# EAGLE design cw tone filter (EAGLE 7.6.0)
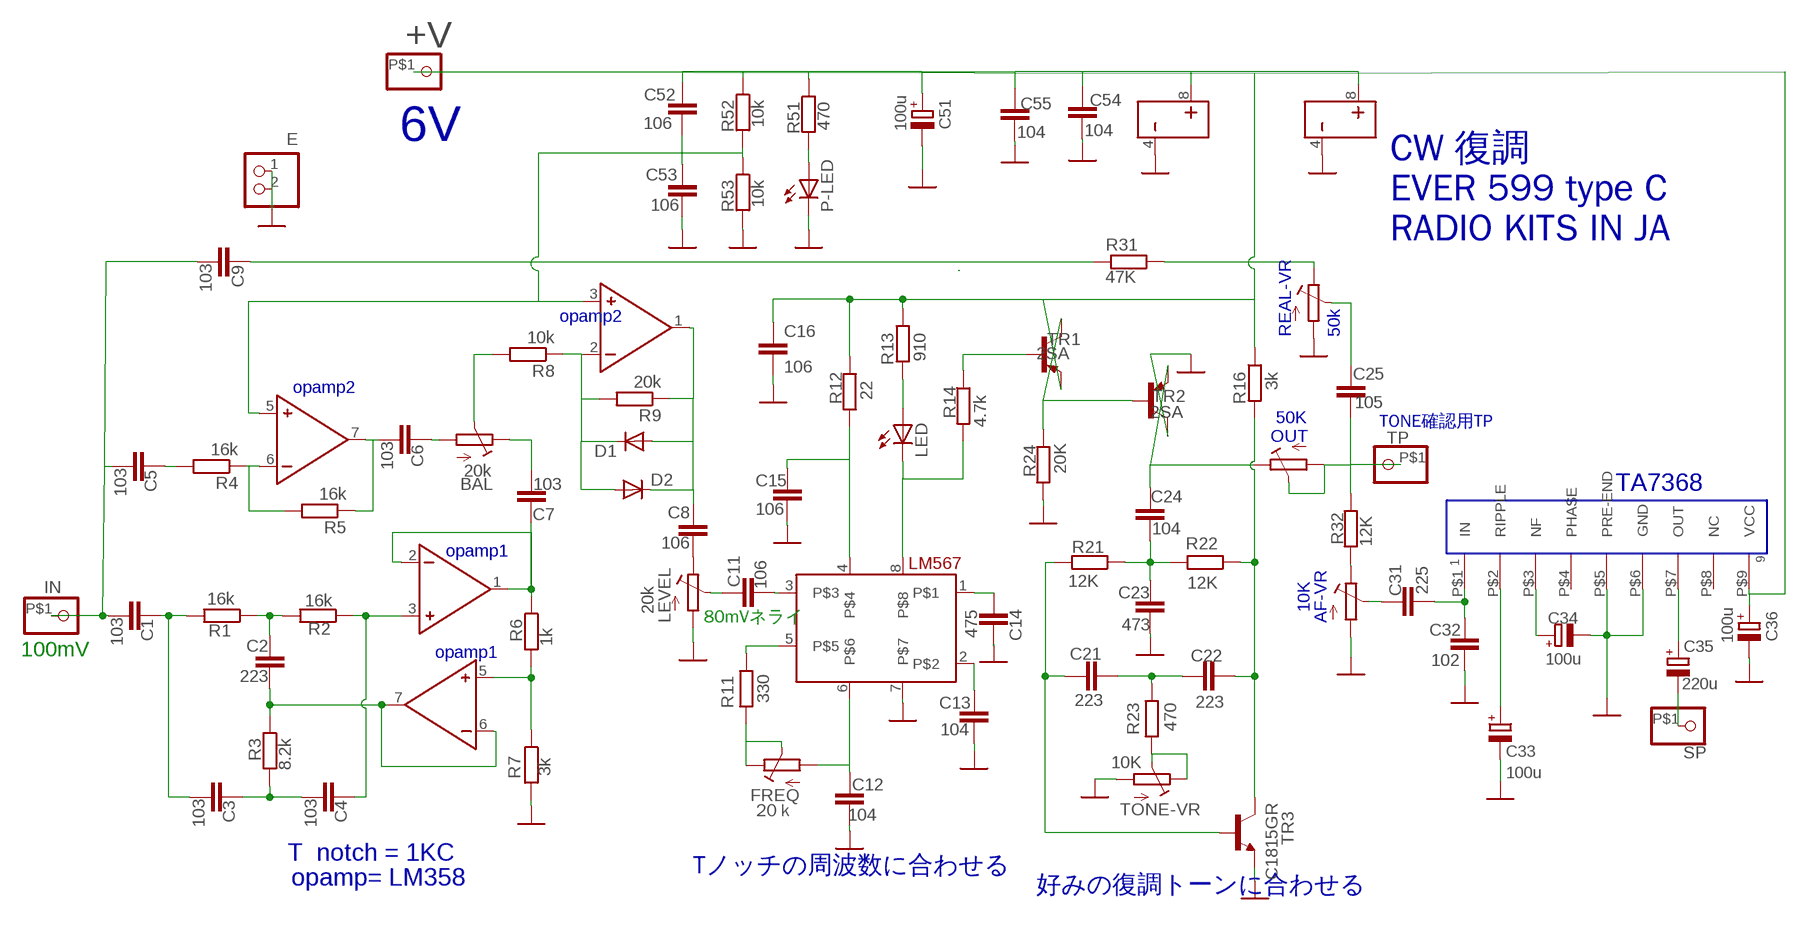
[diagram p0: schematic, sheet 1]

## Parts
+V  PINHD-1X1  [1X01]
AF-VR  10K  SINGLE-VR  [SINGLE-VR]
BAL  20k  R-TRIMM3296W  [RTRIM3296W]
C1  103  C-EU050-024X044  [C050-024X044]
C2  223  C-EU050-024X044  [C050-024X044]
C3  103  C-EU050-024X044  [C050-024X044]
C4  103  C-EU050-024X044  [C050-024X044]
C5  103  C-EU050-024X044  [C050-024X044]
C6  103  C-EU050-024X044  [C050-024X044]
C7  103  C-EU050-024X044  [C050-024X044]
C8  106  C-EU050-024X044  [C050-024X044]
C9  103  C-EU050-024X044  [C050-024X044]
C11  106  C-EU050-024X044  [C050-024X044]
C12  104  C-EU050-024X044  [C050-024X044]
C13  104  C-EU050-024X044  [C050-024X044]
C14  475  C-EU050-024X044  [C050-024X044]
C15  106  C-EU050-024X044  [C050-024X044]
C16  106  C-EU050-024X044  [C050-024X044]
C21  223  C-EU050-024X044  [C050-024X044]
C22  223  C-EU050-024X044  [C050-024X044]
C23  473  C-EU050-024X044  [C050-024X044]
C24  104  C-EU050-024X044  [C050-024X044]
C25  105  C-EU050-024X044  [C050-024X044]
C31  225  C-EU050-024X044  [C050-024X044]
C32  102  C-EU050-024X044  [C050-024X044]
C33  100u  CPOL-EUE2.5-6  [E2,5-6]
C34  100u  CPOL-EUE2.5-6  [E2,5-6]
C35  220u  CPOL-EUE2.5-6  [E2,5-6]
C36  100u  CPOL-EUE2.5-6  [E2,5-6]
C51  100u  CPOL-EUE2.5-6  [E2,5-6]
C52  106  C-EU050-024X044  [C050-024X044]
C53  106  C-EU050-024X044  [C050-024X044]
C54  104  C-EU050-024X044  [C050-024X044]
C55  104  C-EU050-024X044  [C050-024X044]
D1  DIODE-D-5  [D-5]
D2  DIODE-D-5  [D-5]
E  PINHD-1X2  [1X02]
FREQ  20ｋ  R-TRIMM3296W  [RTRIM3296W]
IN  PINHD-1X1  [1X01]
LED  LEDIRL80A  [IRL80A]
LEVEL  20k  R-TRIMM3296W  [RTRIM3296W]
LM567  LM567  [NE612]
OPAMP1  4558  [DIL08]
OPAMP2  4558  [DIL08]
OUT  50K  R-TRIMM3296W  [RTRIM3296W]
P-LED  LEDIRL80A  [IRL80A]
R1  16k  R-EU_0204/5  [0204/5]
R2  16k  R-EU_0204/5  [0204/5]
R3  8.2k  R-EU_0204/5  [0204/5]
R4  16k  R-EU_0204/5  [0204/5]
R5  16k  R-EU_0204/5  [0204/5]
R6  1k  R-EU_0204/5  [0204/5]
R7  3k  R-EU_0204/5  [0204/5]
R8  10k  R-EU_0204/5  [0204/5]
R9  20k  R-EU_0204/5  [0204/5]
R11  330  R-EU_0204/5  [0204/5]
R12  22  R-EU_0204/5  [0204/5]
R13  910  R-EU_0204/5  [0204/5]
R14  4.7k  R-EU_0204/5  [0204/5]
R16  3k  R-EU_0204/5  [0204/5]
R21  12K  R-EU_0204/5  [0204/5]
R22  12K  R-EU_0204/5  [0204/5]
R23  470  R-EU_0204/5  [0204/5]
R24  20K  R-EU_0204/5  [0204/5]
R31  47K  R-EU_0204/5  [0204/5]
R32  12K  R-EU_0204/5  [0204/5]
R51  470  R-EU_0204/5  [0204/5]
R52  10k  R-EU_0204/5  [0204/5]
R53  10k  R-EU_0204/5  [0204/5]
REAL-VR  50k  R-TRIMM3296W  [RTRIM3296W]
SP  PINHD-1X1  [1X01]
TA7368  TA7368P  [TA7368P]
TONE-VR  10K  R-TRIMM3296W  [RTRIM3296W]
TP  PINHD-1X1  [1X01]
TR1  2SA  [TO92-ECB]
TR2  2SA  [TO92-ECB]
TR3  C1815GR  2SC1815  [TO92-ECB]

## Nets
9V: +V.P$1 C16.1 C36.+ C51.+ C52.1 C54.2 C55.2 OPAMP1.8 OPAMP2.8 R12.1 R13.1 R16.1 R51.1 R52.1 TA7368.P$9(VCC) TR1.E
GND: AF-VR.P$3(E) C12.2 C13.2 C14.1 C15.2 C16.2 C23.2 C32.2 C33.- C34.- C36.- C51.- C53.2 C54.1 C55.1 E.1 E.2 LEVEL.1(E) LM567.7 OPAMP1.4 OPAMP2.4 P-LED.K(C) R7.2 R24.2 R53.2 REAL-VR.1(E) TA7368.P$5(PRE-END) TA7368.P$6(GND) TONE-VR.1(E) TR2.C TR3.E
N$1: C8.2 LEVEL.3(A)
N$2: C52.2 C53.1 OPAMP2.3 OPAMP2.5 R52.2 R53.1
N$3: C25.2 REAL-VR.2(S)
N$4: C11.1 LM567.3
N$5: C2.1 R1.1 R2.2
N$6: C13.1 LM567.2
N$7: C3.2 C4.1 R3.2
N$8: C14.2 LM567.1
N$9: C1.2 C3.1 R1.2
N$10: C1.1 C5.1 C9.1 IN.P$1
N$11: LM567.5 R11.1
N$12: C24.1 OUT.3(A) TR2.E
N$13: C31.2 C32.1 TA7368.P$1(IN)
N$14: C35.- SP.P$1
N$15: AF-VR.P$2(S) C31.1
N$16: C35.+ TA7368.P$7(OUT)
N$18: C4.2 OPAMP1.3 R2.1
N$19: AF-VR.P$1(A) R32.2
N$20: C22.2 R16.2 R22.1 TR3.C
N$21: R31.1 REAL-VR.3(A)
N$22: C7.1 OPAMP1.1 OPAMP1.2 R6.1
N$23: OPAMP1.5 R6.2 R7.1
N$24: LED.A R13.2
N$25: C2.2 OPAMP1.6 OPAMP1.7 R3.1
N$27: BAL.1(E) C6.2
N$28: C6.1 OPAMP2.7 R5.1
N$29: C5.2 R4.2
N$30: OPAMP2.6 R4.1 R5.2
N$31: BAL.3(A) C7.2
N$32: BAL.2(S) R8.2
N$33: D1.C D2.A OPAMP2.2 R8.1 R9.2
N$34: C8.1 D1.A D2.C OPAMP2.1 R9.1
N$35: C12.1 FREQ.1(E) LM567.6
N$36: R24.1 TR1.C TR2.B
N$38: R23.1 TONE-VR.2(S) TONE-VR.3(A)
N$39: LED.K(C) LM567.8 R14.2
N$41: C25.1 OUT.1(E) OUT.2(S) R32.1 TP.P$1
N$42: C9.2 R31.2
N$43: C15.1 LM567.4 R12.2
N$44: C21.2 C22.1 R23.2
N$45: C21.1 R21.2 TR3.B
N$46: C11.2 LEVEL.2(S)
N$47: C23.1 C24.2 R21.1 R22.2
N$49: C34.+ TA7368.P$3(NF)
N$50: C33.+ TA7368.P$2(RIPPLE)
N$52: R14.1 TR1.B
N$53: FREQ.2(S) FREQ.3(A) R11.2
N$59: P-LED.A R51.2
Unconnected: TA7368.P$4(PHASE) TA7368.P$8(NC)

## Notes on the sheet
- 6V
- CW 復調　
  EVER 599 type C
  RADIO KITS IN JA
- opamp2
- opamp2
- TONE確認用TP
- opamp1
- 80mVネライ
- 100mV | opamp1
- T  notch = 1KC
- Tノッチの周波数に合わせる
- opamp= LM358
- 好みの復調トーンに合わせる

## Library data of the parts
+V IN SP TP = pinhead:PINHD-1X1: PIN HEADER
AF-VR = resistor:SINGLE-VR
BAL FREQ LEVEL OUT REAL-VR TONE-VR = resistor:R-TRIMM: Trimm resistor
C1-C9 C11-C16 C21-C25 C31 C32 C52-C55 = resistor:C-EU: CAPACITOR, European symbol
C33-C36 C51 = resistor:CPOL-EU: POLARIZED CAPACITOR, European symbol
D1 D2 = diode:DIODE-: DIODE
E = pinhead:PINHD-1X2: PIN HEADER
LED P-LED = led:LED: LED
LM567 = ssm2166 :LM567
OPAMP1 OPAMP2 = ic-package:4558
R1-R9 R11-R14 R16 R21-R24 R31 R32 R51-R53 = resistor:R-EU_: RESISTOR, European symbol
TA7368 = lc7265:TA7368P
TR1 TR2 = transistor:2SA
TR3 = transistor:2SC1815: NPN EPITAXIAL TRANSISTOR Source: TOSHIBA .. 2SC1815 1.pdf

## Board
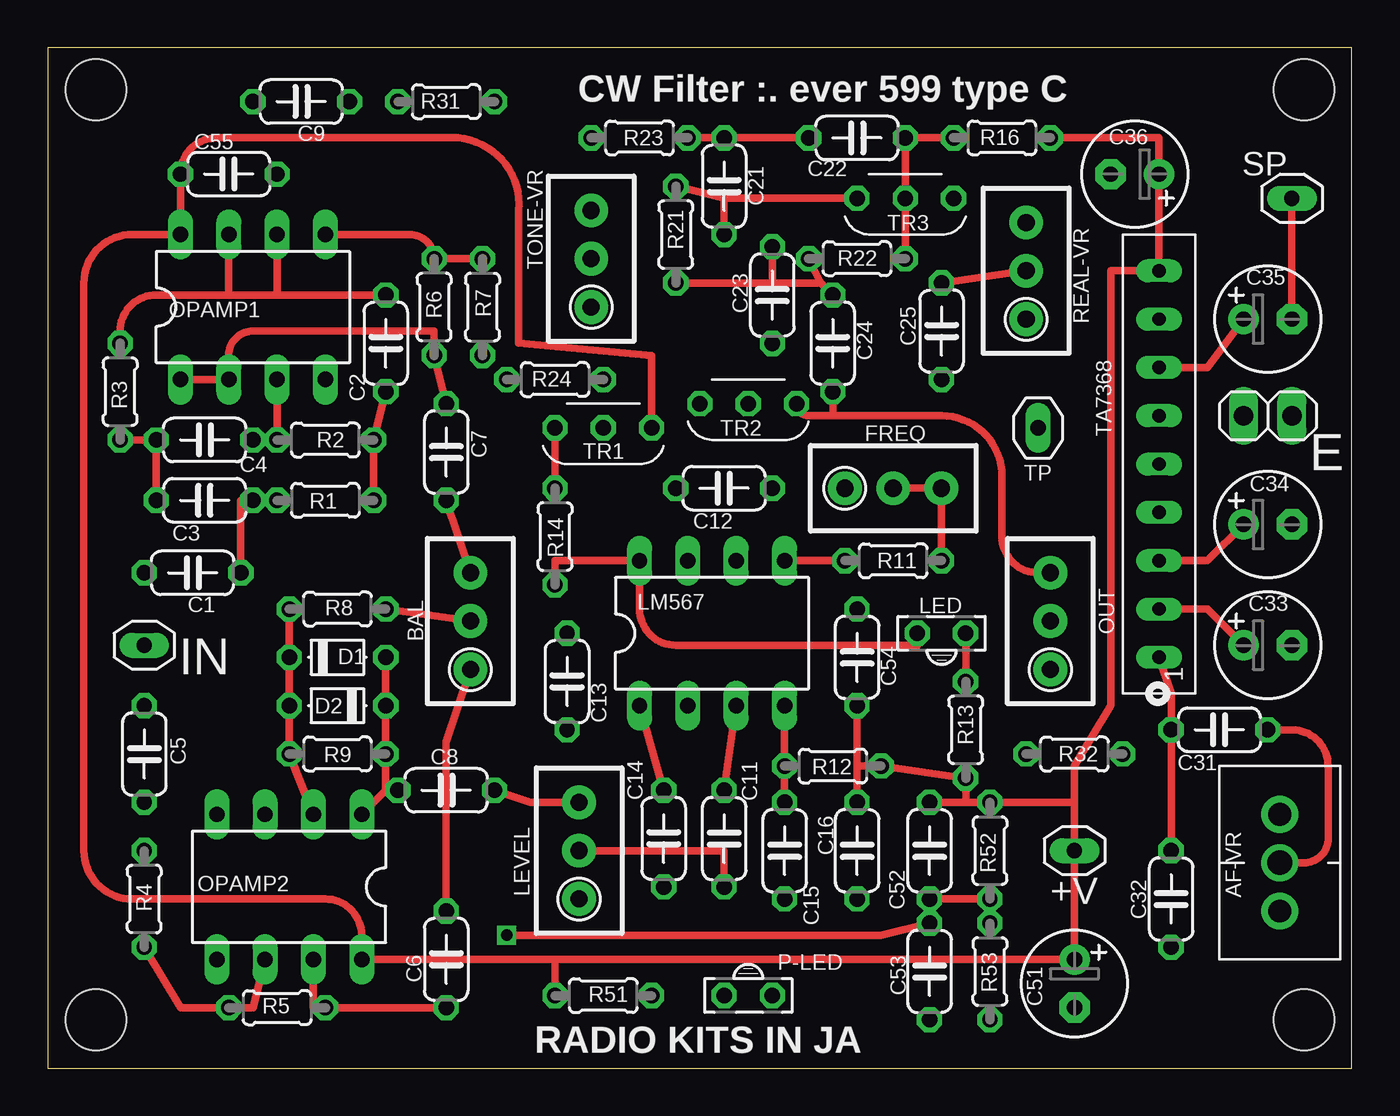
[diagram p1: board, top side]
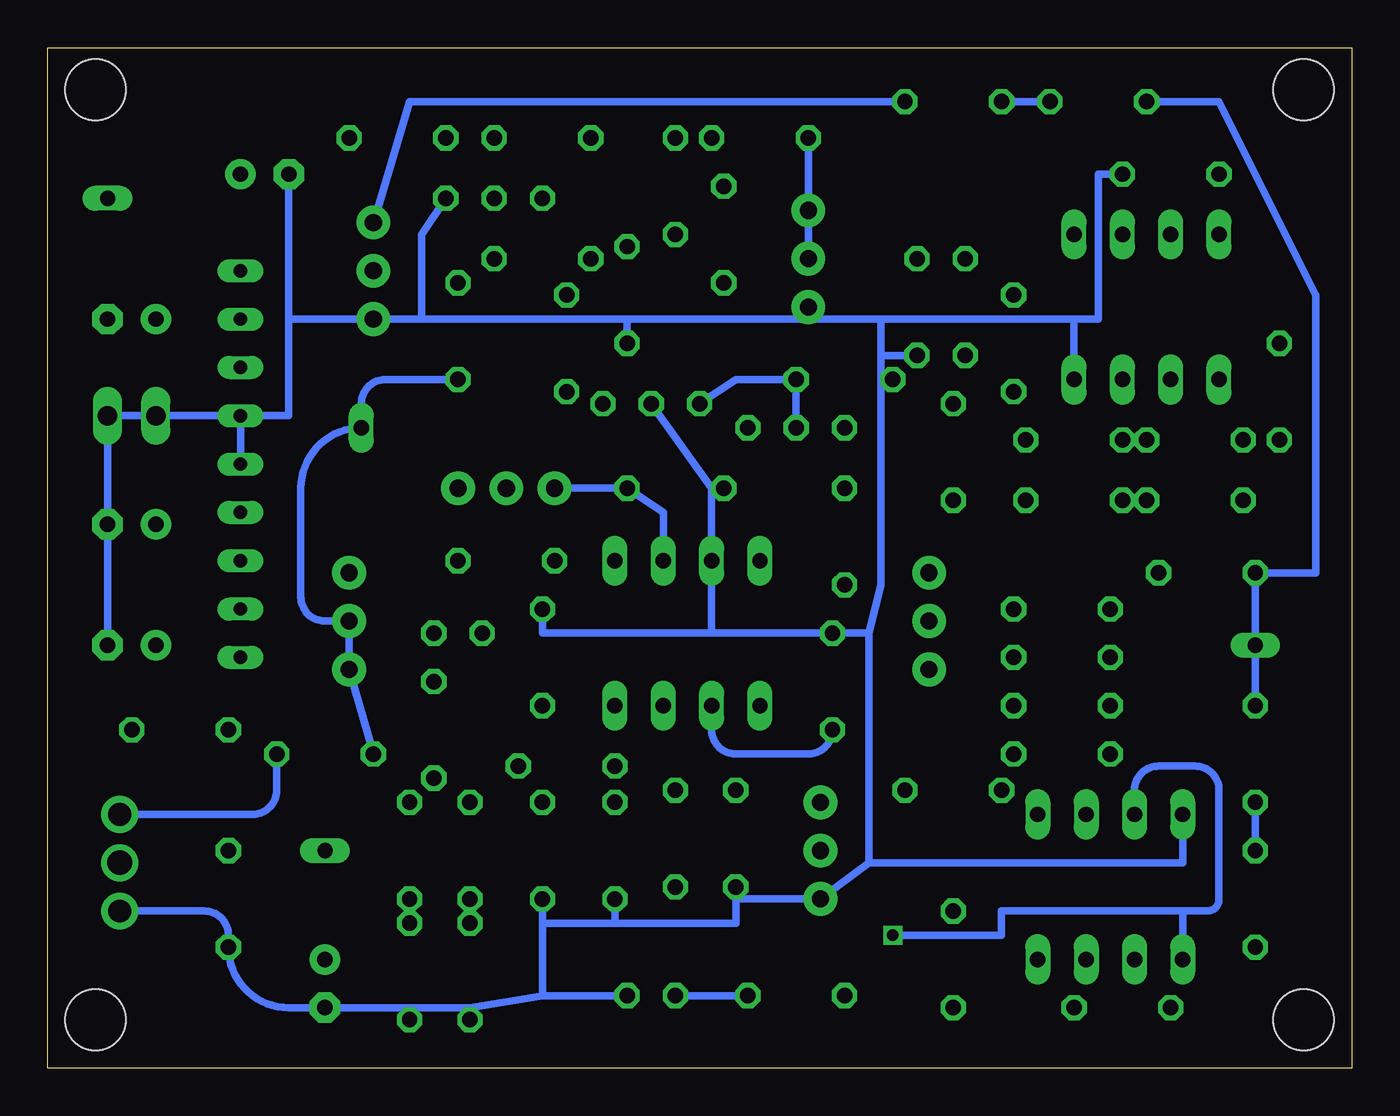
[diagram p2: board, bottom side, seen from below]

Size 68.56 x 53.65 mm. Coordinates in mm from the lower left corner, seen from the top.
Outline: 0,0 68.56,0 68.56,53.65 0,53.65 0,0
Copper layers (1*16): Top 0.035mm / dielectric 1.5mm / Bottom 0.035mm
Design rules "default": minimum track width 10mil, minimum drill 24mil, track to track 8mil, track to pad 8mil, pad to pad 8mil, via to via 8mil, smd to smd 8mil, copper to edge 40mil, drill to drill 8mil, minimum pad ring 10mil, minimum via ring 8mil, stop-mask expansion 4mil, vias tented up to drill 0mil, thermal gap 10mil
Holes 3.2 mm at 66.04,2.54 2.54,51.44 2.54,2.54 66.04,51.44

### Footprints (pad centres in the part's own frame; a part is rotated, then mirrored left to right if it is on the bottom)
1X01 = drill 0.8 long: P$1 0,0
SINGLE-VR = drill 1.2 pad 1.93: P$1 0.635,2.54; P$3 0.635,-2.54 | drill 1.3 pad 1.93: P$2 0.635,0
RTRIM3296W = drill 0.9 pad 1.778: 1 0,-2.54; 2 0,0; 3 0,2.54
C050-024X044 = drill 0.813 octagon: 1 -2.54,0; 2 2.54,0
E2,5-6 = drill 0.813 pad 1.6: + -1.27,0 | drill 0.813 pad 1.6 octagon: - 1.27,0
D-5 = drill 0.813 octagon: A 2.54,0; C -2.54,0
1X02 = drill 1.016 long: 1 -1.27,0; 2 1.27,0
IRL80A = drill 0.813 octagon: A 0,-1.27; K 0,1.27
NE612 = drill 0.813 long: 1 1.27,-3.81; 2 3.81,-3.81; 3 6.35,-3.81; 4 8.89,-3.81; 5 8.89,3.81; 6 6.35,3.81; 7 3.81,3.81; 8 1.27,3.81
DIL08 = drill 0.813 long: 1 -3.81,-3.81; 2 -1.27,-3.81; 3 1.27,-3.81; 4 3.81,-3.81; 5 3.81,3.81; 6 1.27,3.81; 7 -1.27,3.81; 8 -3.81,3.81
0204/5 = drill 0.813 octagon: 1 -2.54,0; 2 2.54,0
TA7368P = drill 0.7 long: P$1 -6.35,1.27; P$2 -3.81,1.27; P$3 -1.27,1.27; P$4 1.27,1.27; P$5 3.81,1.27; P$6 6.35,1.27; P$7 8.89,1.27; P$8 11.43,1.27; P$9 13.97,1.27
TO92-ECB = drill 0.813 octagon: B -2.54,0; C 0,0; E 2.54,0

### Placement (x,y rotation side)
+V  53.98,11.43 0 top
AF-VR  64.13,10.79 0 top
BAL  22.23,23.5 0 top
C1  7.62,26.04 0 top
C2  17.78,38.1 90 top
C3  8.26,29.84 180 top
C4  8.26,33.02 0 top
C5  5.08,16.51 270 top
C6  20.96,5.71 90 top
C7  20.96,32.38 270 top
C8  20.96,14.6 0 top
C9  13.34,50.8 0 top
C11  35.56,12.06 270 top
C12  35.56,30.48 180 top
C13  27.3,20.32 90 top
C14  32.38,12.06 90 top
C15  38.74,11.43 270 top
C16  42.55,11.43 270 top
C21  35.56,46.36 90 top
C22  42.55,48.9 0 top
C23  38.1,40.64 270 top
C24  41.27,38.1 90 top
C25  46.99,38.73 90 top
C31  61.6,17.78 180 top
C32  59.05,8.89 270 top
C33  64.13,22.23 0 top
C34  64.13,28.58 0 top
C35  64.13,39.37 0 top
C36  57.15,46.99 180 top
C51  53.98,4.45 270 top
C52  46.35,11.43 270 top
C53  46.35,5.08 270 top
C54  42.55,21.59 270 top
C55  9.52,46.99 180 top
D1  15.24,21.59 0 top
D2  15.24,19.05 180 top
E  64.13,34.29 0 top
FREQ  44.45,30.48 270 top
IN  5.08,22.23 0 top
LED  46.99,22.86 90 top
LEVEL  27.94,11.43 0 top
LM567  29.85,22.86 0 top
OPAMP1  10.8,40.01 0 top
OPAMP2  12.7,9.53 180 top
OUT  52.71,23.5 0 top
P-LED  36.83,3.81 270 top
R1  14.61,29.84 180 top
R2  14.61,33.02 0 top
R3  3.81,35.56 270 top
R4  5.08,8.89 90 top
R5  12.07,3.17 180 top
R6  20.32,40.01 90 top
R7  22.86,40.01 270 top
R8  15.24,24.13 0 top
R9  15.24,16.51 180 top
R11  44.45,26.67 0 top
R12  41.27,15.87 180 top
R13  48.26,17.78 90 top
R14  26.67,27.94 270 top
R16  50.16,48.9 180 top
R21  33.02,43.82 90 top
R22  42.55,42.55 180 top
R23  31.12,48.9 0 top
R24  26.67,36.2 180 top
R31  20.96,50.8 180 top
R32  53.98,16.51 0 top
R51  29.21,3.81 0 top
R52  49.53,11.43 270 top
R53  49.53,5.08 270 top
REAL-VR  51.43,41.91 0 top
SP  65.41,45.72 0 top
TA7368  59.69,27.94 90 top
TONE-VR  28.57,42.55 0 top
TP  52.07,33.66 90 top
TR1  29.21,33.66 0 top
TR2  36.83,34.93 0 top
TR3  45.09,45.72 0 top

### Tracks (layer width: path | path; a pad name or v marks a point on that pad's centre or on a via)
9V
  Top 0.406: 26.67,5.71 C51.+ +V.P$1 53.98,13.97 | 26.67,5.71 OPAMP2.8 16.51,6.99 arc90 14.61,8.89 4.45,8.89 arc-90 1.91,11.43 1.91,41.27 arc-90 4.45,43.82 OPAMP1.8 C55.2 arc-90 8.89,48.9 21.59,48.9 arc-90 24.77,45.09 24.77,38.1 31.75,37.47 TR1.E | R51.1 26.67,5.71 | 53.98,13.97 53.98,15.87 55.88,19.05 55.88,41.91 TA7368.P$9 C36.+ 58.42,48.9 R16.1 | 53.98,13.97 R52.1 48.26,13.97 | 42.55,15.87 C54.2 | C16.1 42.55,15.87 | 42.55,15.87 R12.1 R13.1 48.26,13.97 | 48.26,13.97 C52.1
GND
  Bottom 0.406: OPAMP1.4 14.61,39.37 | 14.61,39.37 24.77,39.37 | 24.77,39.37 28.57,39.37 | 25.4,10.79 LEVEL.1 32.38,8.89 C14.1 32.38,7.62 38.74,7.62 | 33.66,22.86 LM567.7 33.66,30.48 | 25.4,22.86 C13.2 33.66,22.86 | 25.4,22.86 24.77,25.4 24.77,36.2 | C15.2 38.74,7.62 | C16.2 42.55,7.62 | 42.55,7.62 38.74,7.62 | C55.1 13.34,46.99 13.34,39.37 14.61,39.37 | C54.1 42.55,22.86 33.66,22.86 | 42.55,3.81 42.55,7.62 | P-LED.K 42.55,3.81 | 33.66,30.48 C12.2 | TA7368.P$5 TA7368.P$6 | TA7368.P$6 E.1 E.2 C34.- C33.- | 28.57,39.37 38.1,39.37 | TONE-VR.1 28.57,39.37 | 24.77,37.47 24.77,39.37 | R7.2 24.77,37.47 | 33.66,30.48 TR2.C | C23.2 38.1,39.37 | 38.1,39.37 48.9,39.37 | 48.9,39.37 REAL-VR.1 55.88,39.37 | TR3.E 48.9,43.82 48.9,39.37 | 55.88,39.37 55.88,34.29 TA7368.P$6 | 55.88,39.37 C36.- | OPAMP2.4 8.89,10.79 25.4,10.79 | 42.55,3.81 46.35,3.17 | 46.35,3.17 49.53,3.17 | 49.53,3.17 C51.- 55.88,3.17 arc90 C32.2 59.05,6.99 arc-90 60.32,8.26 AF-VR.P$3 | R53.2 49.53,3.17 | C53.2 46.35,3.17 | 25.4,10.79 25.4,22.86 | 24.77,36.2 24.77,37.47 | R24.2 24.77,36.2
N$1
  Top 0.406: LEVEL.3 25.4,13.97 C8.2
N$2  (via drill 0.6)
  Top 0.406: R53.1 R52.2 C52.2 C53.1 43.82,6.99 v24.13,6.99
  Bottom 0.406: v24.13,6.99 18.41,6.99 18.41,8.26 8.89,8.26 | 8.89,8.26 OPAMP2.5 | 8.89,8.26 7.62,8.26 arc-90 6.98,8.89 6.98,14.6 arc-90 8.26,15.87 10.16,15.87 arc-90 11.43,14.6 OPAMP2.3
N$3
  Top 0.406: REAL-VR.2 C25.2
N$4
  Top 0.406: LM567.3 C11.1
N$5
  Top 0.406: C2.1 R2.2 R1.1
N$6
  Bottom 0.406: C13.1 arc90 28.57,16.51 32.38,16.51 arc90 33.66,17.78 LM567.2
N$7
  Top 0.406: R3.2 C4.1 C3.2
N$8
  Top 0.406: LM567.1 C14.2
N$9
  Top 0.406: R1.2 C3.1 10.16,29.84 C1.2
N$10
  Bottom 0.406: C9.1 6.98,50.8 1.91,40.64 1.91,26.04 C1.1 IN.P$1 C5.1
N$11
  Top 0.406: LM567.5 R11.1
N$12
  Top 0.406: OUT.3 52.07,26.04 arc-90 50.16,27.94 50.16,31.12 arc90 46.99,34.29 41.27,34.29 | 41.27,34.29 40.01,34.29 arc-90 TR2.E | C24.1 41.27,34.29
N$13
  Top 0.406: C32.1 C31.2 59.05,19.69 TA7368.P$1
N$14
  Top 0.406: SP.P$1 C35.-
N$15
  Top 0.406: C31.1 65.41,17.78 arc-90 67.31,15.87 67.31,12.06 arc-90 66.04,10.79 AF-VR.P$2
N$16
  Top 0.406: TA7368.P$7 60.96,36.83 C35.+
N$18
  Top 0.406: OPAMP1.3 R2.1 C4.2
N$19
  Bottom 0.406: AF-VR.P$1 57.79,13.33 arc-90 56.52,14.6 R32.2
N$20
  Top 0.406: R22.1 TR3.C C22.2 R16.2
N$21
  Bottom 0.406: REAL-VR.3 49.53,50.8 R31.1
N$22
  Top 0.406: OPAMP1.1 OPAMP1.2 9.52,37.47 arc-90 10.8,38.73 20.32,38.73 R6.1 C7.1
N$23
  Top 0.406: OPAMP1.5 19.05,43.82 arc-90 R6.2 R7.1
N$24
  Top 0.406: LED.A R13.2
N$25
  Top 0.406: 9.52,40.64 12.07,40.64 | 12.07,40.64 C2.2 | R3.1 3.81,38.73 arc-90 5.72,40.64 9.52,40.64 | 9.52,40.64 OPAMP1.7 | OPAMP1.6 12.07,40.64
N$27
  Top 0.406: BAL.1 20.96,17.15 C6.2
N$28
  Top 0.406: OPAMP2.7 13.97,3.17 R5.1 C6.1
N$29
  Bottom 0.406: R4.2 C5.2
N$30
  Top 0.406: OPAMP2.6 10.8,3.17 R5.2 6.98,3.17 R4.1
N$31
  Top 0.406: C7.2 BAL.3
N$32
  Top 0.406: R8.2 BAL.2
N$33
  Top 0.406: R8.1 D1.C D2.A R9.2 OPAMP2.2
N$34
  Top 0.406: D1.A D2.C R9.1 17.78,14.6 | 17.78,14.6 OPAMP2.1 | C8.1 17.78,14.6
N$35
  Bottom 0.406: FREQ.1 C12.1 36.2,29.21 LM567.6
N$36
  Bottom 0.406: TR1.C R24.1 32.38,36.2 TR2.B
N$38
  Bottom 0.406: TONE-VR.2 TONE-VR.3 R23.1
N$39
  Top 0.406: LED.K 45.72,22.23 33.02,22.23 arc-90 31.12,24.13 LM567.8 26.67,26.67 R14.2
N$41
  Bottom 0.406: R32.1 OUT.1 OUT.2 53.98,23.5 arc90 55.24,24.77 55.24,30.48 arc90 TP.P$1 52.07,34.93 arc90 50.8,36.2 C25.1
N$42
  Bottom 0.406: C9.2 R31.2
N$43
  Top 0.406: LM567.4 R12.2 C15.1
N$44
  Top 0.406: C22.1 C21.2 R23.2
N$45
  Top 0.406: R21.2 35.56,45.72 | 35.56,45.72 TR3.B | C21.1 35.56,45.72
N$46
  Top 0.406: C11.2 35.56,11.43 LEVEL.2
N$47
  Top 0.406: R21.1 38.1,41.27 | 38.1,41.27 40.64,41.27 | C23.1 38.1,41.27 | 40.64,41.27 R22.2 | C24.2 40.64,41.27
N$49
  Top 0.406: TA7368.P$3 60.96,26.67 C34.+
N$50
  Top 0.406: TA7368.P$2 60.96,24.13 C33.+
N$52
  Top 0.406: TR1.B R14.1
N$53
  Top 0.406: R11.2 FREQ.3 FREQ.2
N$59
  Bottom 0.406: P-LED.A R51.2

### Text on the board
tNames: CW Filter :. ever 599 type C | RADIO KITS IN JA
